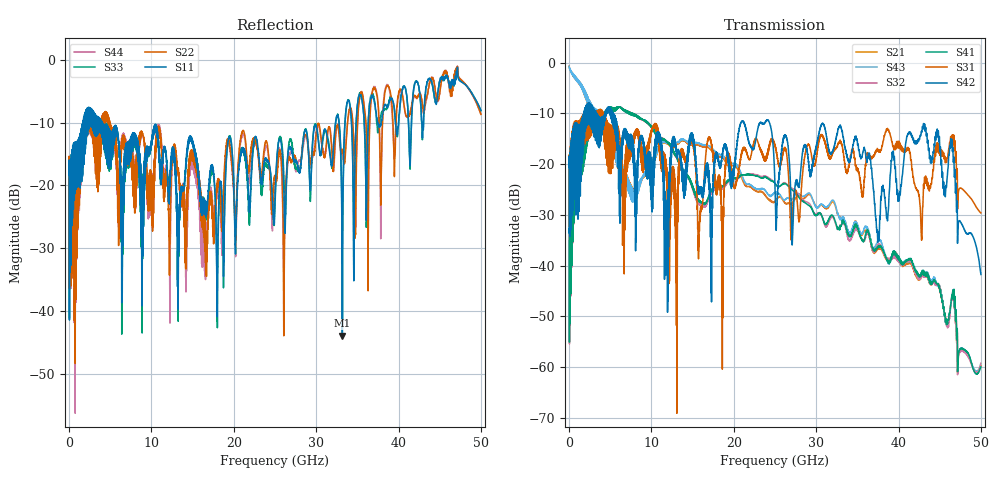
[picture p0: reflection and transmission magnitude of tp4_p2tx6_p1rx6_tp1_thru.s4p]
! 100G CR Analysis
! File: tp4_p2tx6_p1rx6_tp1_thru
! Description: 2m Cu Cable, OSFP, TP1-TP4
! Port Mapping
! Port1 -- P1RX6N
! Port2 -- P2TX6N
! Port3 -- P1RX6P
! Port4 -- P2TX6P
# GHz S MA R 50.00
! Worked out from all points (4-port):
!   5000 points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, 10 MHz to 50 GHz, reference 50 ohm
!   strongest paths, dB at 10 MHz, 12.51 GHz, 25.01 GHz, 37.51 GHz, 50 GHz:
!     S42: -20.7, -15.3, -24.9, -34.8, -41.8
!     S31: -20.5, -20.7, -16.6, -17.4, -29.6
!     S41: -33.4, -17.0, -23.8, -36.4, -60.0
!     S32: -33.5, -17.1, -23.9, -36.0, -59.3
!     S43: -0.7, -16.5, -25.5, -35.3, -59.4
!     S21: -0.7, -16.8, -27.3, -36.8, -59.7
!   lowest |S11| = -43.9 dB at 33.18 GHz (marker M1), VSWR 1.01, Z = 49.8 - j0.618 ohm
!   |S11| at or under -10 dB: start of sweep to 1.667 GHz; 4.032 GHz to 32.35 GHz (28.32 GHz wide, 156 % of centre); 32.78 GHz to 33.5 GHz (719.5 MHz wide, 2.17 % of centre)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
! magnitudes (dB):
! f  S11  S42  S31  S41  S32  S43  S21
! 10 MHz  -18.4  -20.7  -20.5  -33.4  -33.5  -0.7  -0.7
! 6.1 GHz  -14.1  -17.5  -14.3  -8.8  -8.8  -20.7  -20.8
! 15.81 GHz  -20.6  -25.9  -32.3  -27.5  -28.1  -15.9  -16.2
! 33.18 GHz  -43.9  -13.5  -16.5  -31.1  -31.1  -30.4  -30.4
! 37.47 GHz  -10.2  -35.1  -17.3  -36.5  -36.0  -35.4  -36.8
! 46.38 GHz  -3.4  -16.2  -15.9  -47.2  -47.4  -47.2  -47.2
! 50 GHz  -8.1  -41.8  -29.6  -60.0  -59.3  -59.4  -59.7
